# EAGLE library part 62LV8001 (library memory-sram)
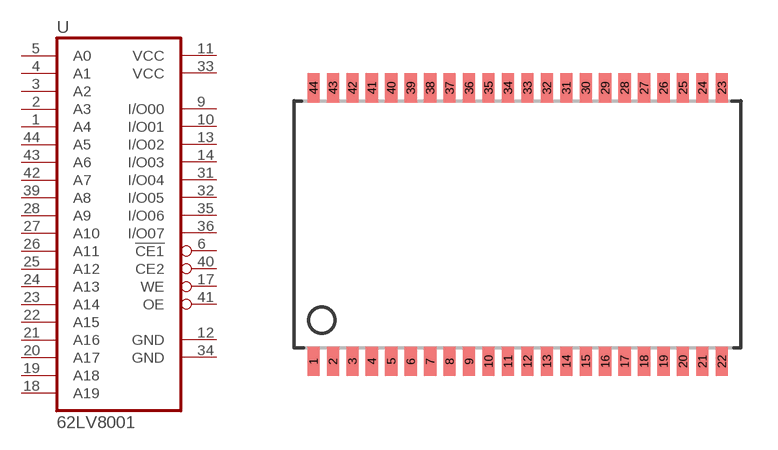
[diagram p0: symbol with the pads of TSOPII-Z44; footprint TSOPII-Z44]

Designator prefix -

## 62LV8001  [TSOPII-Z44]
1  A4  in
2  A3  in
3  A2  in
4  A1  in
5  A0  in
6  !CE1  in
9  I/O00
10  I/O01
11  VCC  pwr
12  GND  pwr
13  I/O02
14  I/O03
17  WE  in
18  A19  in
19  A18  in
20  A17  in
21  A16  in
22  A15  in
23  A14  in
24  A13  in
25  A12  in
26  A11  in
27  A10  in
28  A9  in
31  I/O04
32  I/O05
33  VCC  pwr
34  GND  pwr
35  I/O06
36  I/O07
39  A8  in
40  CE2  in
41  OE  in
42  A7  in
43  A6  in
44  A5  in

## Footprint TSOPII-Z44 (pad centres in mm)
44 PIN TSOP II Z44 Source: CYPRESS cy7c1049cv33_8.pdf
smd 0.5 x 1.2: 1 -8.4,-5.627; 2 -7.6,-5.627; 3 -6.8,-5.627; 4 -6,-5.627; 5 -5.2,-5.627; 6 -4.4,-5.627; 7 -3.6,-5.627; 8 -2.8,-5.627; 9 -2,-5.627; 10 -1.2,-5.627; 11 -0.4,-5.627; 12 0.4,-5.627; 13 1.2,-5.627; 14 2,-5.627; 15 2.8,-5.627; 16 3.6,-5.627; 17 4.4,-5.627; 18 5.2,-5.627; 19 6,-5.627; 20 6.8,-5.627; 21 7.6,-5.627; 22 8.4,-5.627; 23 8.4,5.627; 24 7.6,5.627; 25 6.8,5.627; 26 6,5.627; 27 5.2,5.627; 28 4.4,5.627; 29 3.6,5.627; 30 2.8,5.627; 31 2,5.627; 32 1.2,5.627; 33 0.4,5.627; 34 -0.4,5.627; 35 -1.2,5.627; 36 -2,5.627; 37 -2.8,5.627; 38 -3.6,5.627; 39 -4.4,5.627; 40 -5.2,5.627; 41 -6,5.627; 42 -6.8,5.627; 43 -7.6,5.627; 44 -8.4,5.627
